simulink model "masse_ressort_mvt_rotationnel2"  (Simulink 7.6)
settings: Solver=ode15s  StartTime=0.0  StopTime=0.5  RelTol=1e-3
StopFcn:
  | % lecture du fichier binaire
  | load masse_ressort3.mat
  | 
  | % trace de la tension et du courant d’induit
  | plotyy(x(1,:),x(2,:),x(1,:),x(3,:))
  | title('Position et vitesse linéaire - Régime forcé, réponseà échelon de couple')
  | grid
libraries: fl_lib x8, nesl_utility x4

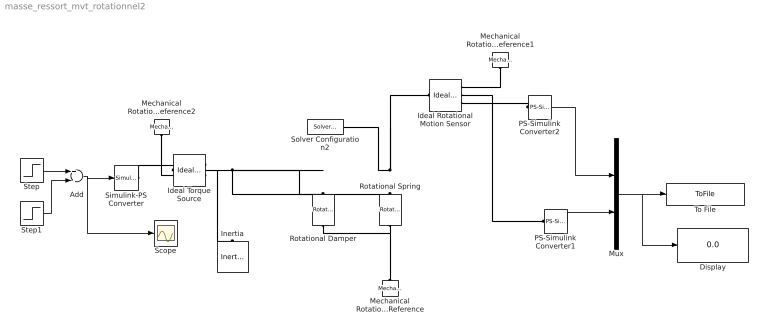
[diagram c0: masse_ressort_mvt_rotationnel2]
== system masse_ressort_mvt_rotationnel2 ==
  Add : Sum  Inputs=+-
  Display : Display
  Ideal Rotational Motion Sensor : fl_lib/Mechanical/Mechanical Sensors/Ideal Rotational Motion Sensor  DialogController=NetworkEngine.DynNeDlgSource  SystemSampleTime=-1  offset=0 rad  w_Log=off  t_Log=off  phi_Log=off  LocalVarNames=|w|t|phi  LocalVarDescs=|w|t|phi  LocalVarLogging=[0 0 0]
  Ideal Torque Source : fl_lib/Mechanical/Mechanical Sources/Ideal Torque Source  DialogController=NetworkEngine.DynNeDlgSource  SystemSampleTime=-1  w_Log=off  t_Log=off  LocalVarNames=|w|t  LocalVarDescs=|w|t  LocalVarLogging=[0 0]
  Inertia : fl_lib/Mechanical/Rotational Elements/Inertia  DialogController=NetworkEngine.DynNeDlgSource  SystemSampleTime=-1  inertia=0.001 kg*m^2  initial_velocity=0 rad/s  t_Log=off  LocalVarNames=|t  LocalVarDescs=|t  LocalVarLogging=0
  Mechanical Rotational Reference : fl_lib/Mechanical/Rotational Elements/Mechanical Rotational Reference  DialogController=NetworkEngine.DynNeDlgSource  SystemSampleTime=-1  t_Log=off  LocalVarNames=|t  LocalVarDescs=|t  LocalVarLogging=0
  Mechanical Rotational Reference1 : fl_lib/Mechanical/Rotational Elements/Mechanical Rotational Reference  DialogController=NetworkEngine.DynNeDlgSource  SystemSampleTime=-1  t_Log=off  LocalVarNames=|t  LocalVarDescs=|t  LocalVarLogging=0
  Mechanical Rotational Reference2 : fl_lib/Mechanical/Rotational Elements/Mechanical Rotational Reference  DialogController=NetworkEngine.DynNeDlgSource  SystemSampleTime=-1  t_Log=off  LocalVarNames=|t  LocalVarDescs=|t  LocalVarLogging=0
  Mux : Mux  Inputs=2
  PS-Simulink Converter1 : nesl_utility/PS-Simulink Converter  DialogController=NetworkEngine.DynNeUtilDlgSource  SystemSampleTime=-1  PhysicalDomain=network_engine_domain  LeftPortType=input  RightPortType=output  SubClassName=ps_output  Unit=1  AffineConversion=off
  PS-Simulink Converter2 : nesl_utility/PS-Simulink Converter  DialogController=NetworkEngine.DynNeUtilDlgSource  SystemSampleTime=-1  PhysicalDomain=network_engine_domain  LeftPortType=input  RightPortType=output  SubClassName=ps_output  Unit=1  AffineConversion=off
  Rotational Damper : fl_lib/Mechanical/Rotational Elements/Rotational Damper  DialogController=NetworkEngine.DynNeDlgSource  SystemSampleTime=-1  D=0.1 N*m/(rad/s)  t_Log=off  w_Log=off  LocalVarNames=|t|w  LocalVarDescs=|t|w  LocalVarLogging=[0 0]
  Rotational Spring : fl_lib/Mechanical/Rotational Elements/Rotational Spring  DialogController=NetworkEngine.DynNeDlgSource  SystemSampleTime=-1  spr_rate=10 N*m/rad  init_def=0 rad  t_Log=off  w_Log=off  phi_Log=off  LocalVarNames=|t|w|phi  LocalVarDescs=|t|w|phi  LocalVarLogging=[0 0 0]
  Scope : Scope
  Simulink-PS Converter : nesl_utility/Simulink-PS Converter  DialogController=NetworkEngine.DynNeUtilDlgSource  SystemSampleTime=-1  PhysicalDomain=network_engine_domain  LeftPortType=input  RightPortType=output  SubClassName=ps_input  Unit=1  AffineConversion=off  InputFilterTimeConstant=.001  UdotUserProvided=0
  Solver Configuration2 : nesl_utility/Solver Configuration  DialogController=NetworkEngine.DynNeUtilDlgSource  SystemSampleTime=-1  PhysicalDomain=network_engine_domain  LeftPortType=input  RightPortType=generic  SubClassName=solver  Accelerate=off  Profile=off  ResidualTolerance=1e-9  MaxNonlinIter=12  MaxModeIter=2  DoFixedCost=off  UseLocalSampling=off  DoDC=off  LinearAlgebra=Sparse  LocalSolverSampleTime=.001  LocalSolverChoice=NE_BACKWARD_EULER_ADVANCER  UseLocalSolver=off
  Step : Step  Time=0.1  SampleTime=0
  Step1 : Step  Time=0.3  SampleTime=0
  To File : ToFile  Filename=masse_ressort3.mat  MatrixName=x
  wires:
  PS-Simulink Converter2/1 -> Mux/1
  Mux/1 -> To File/1, Display/1
  PS-Simulink Converter1/1 -> Mux/2
  Step/1 -> Add/1
  Step1/1 -> Add/2
  Add/1 -> Simulink-PS Converter/1, Scope/1
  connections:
  PS-Simulink Converter2/LConn1 -- Ideal Rotational Motion Sensor/RConn3
  Rotational Damper/RConn1 -- Mechanical Rotational Reference/LConn1 -- Rotational Spring/RConn1
  Ideal Rotational Motion Sensor/RConn2 -- PS-Simulink Converter1/LConn1
  Ideal Torque Source/LConn1 -- Solver Configuration2/RConn1 -- Ideal Rotational Motion Sensor/LConn1 -- Rotational Spring/LConn1 -- Rotational Damper/LConn1 -- Inertia/LConn1
  Mechanical Rotational Reference1/LConn1 -- Ideal Rotational Motion Sensor/RConn1
  Simulink-PS Converter/RConn1 -- Ideal Torque Source/RConn1
  Mechanical Rotational Reference2/LConn1 -- Ideal Torque Source/RConn2
